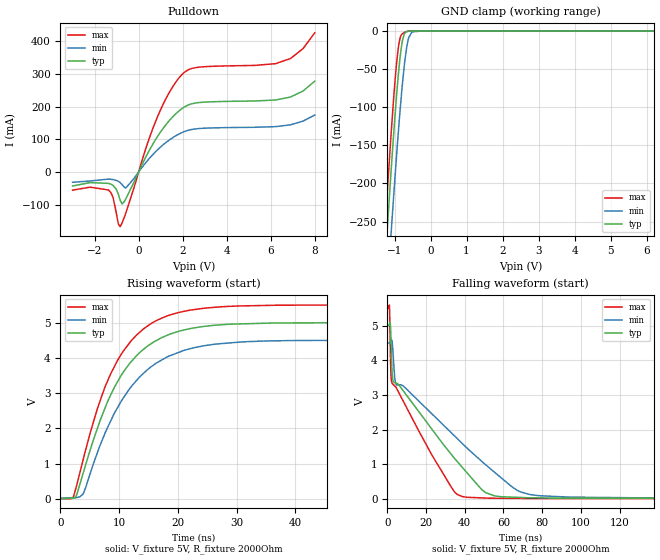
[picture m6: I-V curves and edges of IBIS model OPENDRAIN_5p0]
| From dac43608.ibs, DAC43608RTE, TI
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|   OPENDRAIN_5p0 Model
[Model]   OPENDRAIN_5p0
Model_type   I/O_open_drain
Polarity   Non-Inverting
Enable   Active-Low
Vinl = 0.5
Vinh = 2.4
Vmeas = 2.5
Vref = 5
Cref = 2pF
Rref = 2000
|   typ   min   max
C_comp   1.041E-12   1.022E-12   1.061E-12
|  Where Nom  PVT is Nominal Process, 5.0V,   25C
|   Fast PVT is Strong Process,  5.5V,  -40C
|   Slow PVT is Weak Process,   4.5V,  125C
[Voltage Range]   5   4.5   5.5
|Junction Temperature
[Temperature Range]   25   125   -40
[Pullup Reference]   5   4.5   5.5
[Pulldown Reference]   0   0   0
[Power Clamp Reference]   5   4.5   5.5
[GND Clamp Reference]   0   0   0
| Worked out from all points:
|   slope of the pulldown table from 0 to 0.75 V, typ, clamps not added: 7.74 ohm
|   GND clamp passes 1 mA (typ) near -0.67 V on its own axis
|   falling waveform, V_fixture 5V, R_fixture 2000Ohm: 20-80 % time 35ns typ, 48.6ns min, 23.3ns max; typ from 5 V to 0.017 V
|   rising waveform, V_fixture 5V, R_fixture 2000Ohm: 20-80 % time 8.28ns typ, 8.97ns min, 7.82ns max; typ from 0.017 V to 5 V
[Pulldown]
|   Voltage   I(typ)   I(min)   I(max)
-3V       -42.86mA   -31.34mA   -55.38mA
-1.372V   -34.69mA   -21.67mA   -54.81mA
-1.163V   -40.81mA   -23.12mA   -77.68mA
-833mV    -87.13mA   -32.75mA   -166.3mA
-580mV    -81.83mA   -48.64mA   -125.1mA
740mV     95.82mA    59.81mA    149.2mA
1.356V    154mA      95.98mA    238.5mA
1.983V    194.4mA    120.8mA    298.6mA
2.742V    212.1mA    132.7mA    320.1mA
6.218V    219.9mA    138.5mA    330.9mA
6.911V    229.5mA    144.4mA    347.2mA
8V        277.4mA    174mA      425.1mA
[GND Clamp]
|   Voltage   I(typ)   I(min)   I(max)
-3V       -1.649A    -1.642A    -1.661A
-1.339V   -363mA     -440.9mA   -317.8mA
-1.185V   -248mA     -328.9mA   -200.1mA
-1.086V   -177.3mA   -259mA     -129mA
-998mV    -118.4mA   -199.2mA   -72.22mA
-921mV    -72.04mA   -149.5mA   -32.41mA
-866mV    -43.76mA   -116.1mA   -13.62mA
-811mV    -21.67mA   -85.11mA   -5.256mA
-723mV    -3.389mA   -43.04mA   -1.781mA
-613mV    -216.3uA   -10.15mA   -266.7uA
-514mV    -18.89uA   -1.076mA   -21.66uA
8V        0A         0A         0A
[POWER Clamp]
|   Voltage   I(typ)   I(min)   I(max)
-3V       0A         0A         0A
0V        0A         0A         0A
8V        0A         0A         0A
[Ramp]
R_load = 2000
|   typ   min   max
dV/dt_r   2.98997/8.25972e-09   2.68553/8.9474e-09   3.29296/7.80264e-09
dV/dt_f   2.98997/3.49987e-08   2.68553/4.86978e-08   3.29296/2.31848e-08
[Falling Waveform]
V_fixture = 5V
V_fixture_min = 4.5V
V_fixture_max = 5.5V
R_fixture = 2000Ohm
C_fixture = 0F
|   Time   V(typ)   V(min)   V(max)
0s        5V         4.5V       5.5V
1.084ns   5.046V     4.502V     5.582V
1.766ns   4.802V     4.559V     3.752V
2.449ns   3.673V     4.555V     3.345V
4.456ns   3.349V     3.317V     3.225V
32.99ns   1.295V     1.916V     352mV
38.8ns    912mV      1.6V       73.15mV
50.75ns   186.3mV    993.1mV    30.14mV
78.54ns   34.78mV    97.48mV    16.27mV
500ns     16.72mV    24.11mV    11.72mV
[Rising Waveform]
V_fixture = 5V
V_fixture_min = 4.5V
V_fixture_max = 5.5V
R_fixture = 2000Ohm
C_fixture = 0F
|   Time   V(typ)   V(min)   V(max)
0s        16.72mV    24.11mV    11.72mV
2.178ns   26.72mV    34.51mV    56.57mV
2.745ns   113.2mV    40.06mV    375.1mV
3.82ns    705mV      139.3mV    1.083V
6.252ns   1.981V     1.297V     2.538V
7.828ns   2.675V     1.955V     3.268V
12.06ns   3.894V     3.186V     4.486V
18.29ns   4.647V     4.036V     5.194V
27.25ns   4.936V     4.402V     5.446V
500ns     5V         4.5V       5.5V
